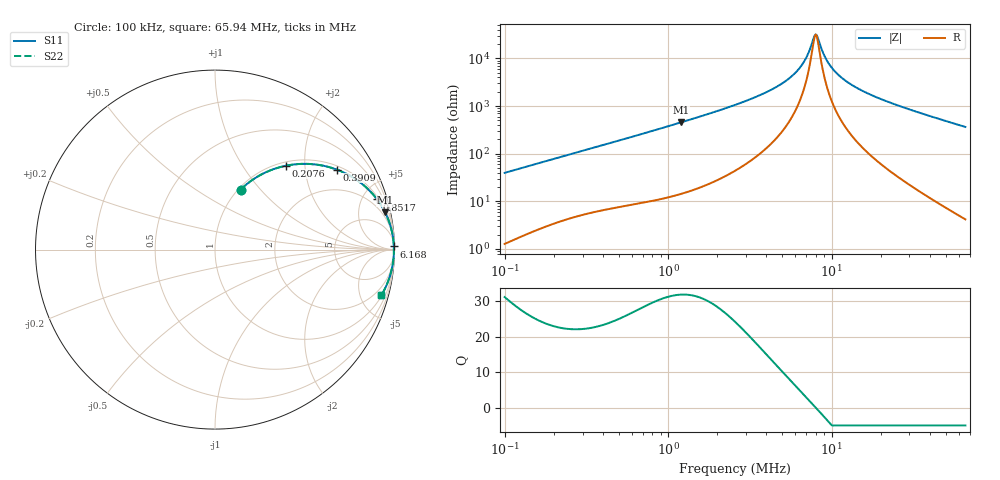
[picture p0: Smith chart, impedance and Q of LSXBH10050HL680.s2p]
! LSXBH10050HL680  S-PARAMETER MODEL  ( General Type )
! Model Generated by TAIYO YUDEN Corporation (http://www.ty-top.com)
! Version 3.0
! TAIYO YUDEN Control No. 180118NI43SB-FBB
! Copyright(c) 2007 TAIYO YUDEN CO.,LTD. All Rights Reserved.
! Product Description (link to TY-COMPAS)
! https://ds.yuden.co.jp/TYCOMPAS/or/detail?pn=LSXBH10050HL680M&u=M
! Products Name : Inductors
! Characteristics :
!  Inductance : 68 uH , SRF(min) : 5.6 MHz , DC Resistance(max) : 0.1872 Ohm
!  Rated Current : Saturation :1700 mA , Temp Rise : 1500 mA (40 degC)
!  Case Size : 10.0 x 9.8 / 0.394 x 0.386 [mm/inch] , Thickness : 5 / 0.197 [mm/inch]
!  (Conditions: Temperature = 25 degC , DC Bias Current/Voltage = 0A / 0V)
! External Node Assignments :
!  1  o---GGG---o  2
! GND o---------o GND
! Frequency Range : 0.1MHz  -  65.935307MHz  [ 402 STEP ]
# MHz S RI R 50
! Freq[MHz].  S11 Real  S11 Imag  S21 Real  S21 Imag  S12 Real  S12 Imag  S22 Real  S22 Imag
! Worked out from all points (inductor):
!   401 points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, 100 kHz to 65.94 MHz, reference 50 ohm
!   read as one part in series: L = 62.6 uH near 103.3 kHz
!   highest Q = 31.8 at 1.198 MHz (marker M1), where L = 60.1 uH
!   self-resonance near 7.997 MHz
!   S11 on the Smith chart (normalised r, x): 100 kHz: 1.03, +0.79; 207.6 kHz: 1.07, +1.61; 390.9 kHz: 1.13, +2.96; 851.7 kHz: 1.21, +6.39; 6.168 MHz: open; 65.94 MHz: 1.08, -7.28
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0.1  0.1431 0.3345  0.8569 -0.3345  0.8569 -0.3345  0.1431 0.3345
0.207563  0.3971 0.4678  0.6029 -0.4678  0.6029 -0.4678  0.3971 0.4678
0.296621  0.5596 0.4743  0.4404 -0.4743  0.4404 -0.4743  0.5596 0.4743
0.390854  0.6792 0.4456  0.3208 -0.4456  0.3208 -0.4456  0.6792 0.4456
0.851744  0.9031 0.2796  0.0969 -0.2796  0.0969 -0.2796  0.9031 0.2796
0.879842  0.9085 0.2723  0.0915 -0.2723  0.0915 -0.2723  0.9085 0.2723
1.197602  0.9475 0.2078  0.0525 -0.2078  0.0525 -0.2078  0.9475 0.2078
2.609798  0.9877 0.0914  0.0123 -0.0914  0.0123 -0.0914  0.9877 0.0914
4.458452  0.9949 0.0417  0.00507 -0.0417  0.00507 -0.0417  0.9949 0.0417
5.329786  0.996 0.0282  0.00404 -0.0282  0.00404 -0.0282  0.996 0.0282
6.167937  0.9965 0.0178  0.00351 -0.0178  0.00351 -0.0178  0.9965 0.0178
6.909944  0.9967 0.01  0.00326 -0.01  0.00326 -0.01  0.9967 0.01
7.616602  0.9969 0.00342  0.00315 -0.00342  0.00315 -0.00342  0.9969 0.00342
7.867865  0.9969 0.00123  0.00313 -0.00123  0.00313 -0.00123  0.9969 0.00123
8.127416  0.9969 -0.000953  0.00312 0.000953  0.00312 0.000953  0.9969 -0.000953
8.958581  0.9968 -0.00752  0.00316 0.00752  0.00316 0.00752  0.9968 -0.00752
9.559395  0.9968 -0.0119  0.00324 0.0119  0.00324 0.0119  0.9968 -0.0119
10.53701  0.9966 -0.0187  0.00344 0.0187  0.00344 0.0187  0.9966 -0.0187
11.80461  0.9962 -0.0267  0.00379 0.0267  0.00379 0.0267  0.9962 -0.0267
15.30441  0.9948 -0.0466  0.00524 0.0466  0.00524 0.0466  0.9948 -0.0466
22.59246  0.9901 -0.0824  0.00992 0.0824  0.00992 0.0824  0.9901 -0.0824
65.93531  0.9273 -0.2539  0.0727 0.2539  0.0727 0.2539  0.9273 -0.2539
